(* Logix 5000 AddOnInstructionDefinition export Bronkhorst_Extended_INT_Input; software revision 37.00 *)

ADD_ON_INSTRUCTION Bronkhorst_Extended_INT_Input   (* revision 1.0, vendor Bronkhorst High-Tech B.V. *)
// Extract data from the Extended INT input connection (in to controller from device)
VAR_IN_OUT
   DataIn : SINT[8]; {required}
END_VAR
VAR_OUTPUT
   Status : SINT; {visible}
   Measure : INT; {visible}
   Setpoint : INT; {visible}
   Override : USINT; {visible}
   Actuator : UINT; {visible}
END_VAR

ROUTINE Logic   (* structured text *)
   Status := DataIn[0];
   COP(DataIn[1], Measure, 1);
   COP(DataIn[3], Setpoint, 1);
   Override := DataIn[5];
   COP(DataIn[6], Actuator , 1);
END_ROUTINE
END_ADD_ON_INSTRUCTION

ADD_ON_INSTRUCTION Bronkhorst_Extended_INT_Output   (* revision 1.0, vendor Bronkhorst High-Tech B.V. *)
// Fill data for the Extended INT output connection (out from controller to device)
VAR_IN_OUT
   DataOut : SINT[3]; {required}   // SINT device output data array
END_VAR
VAR_INPUT
   Override : USINT; {visible}
   Setpoint : INT; {visible}   // INT Setpoint
END_VAR

ROUTINE Logic   (* structured text *)
   DataOut[0] := Override;
   COP(Setpoint, DataOut[1], 2);
END_ROUTINE
END_ADD_ON_INSTRUCTION
